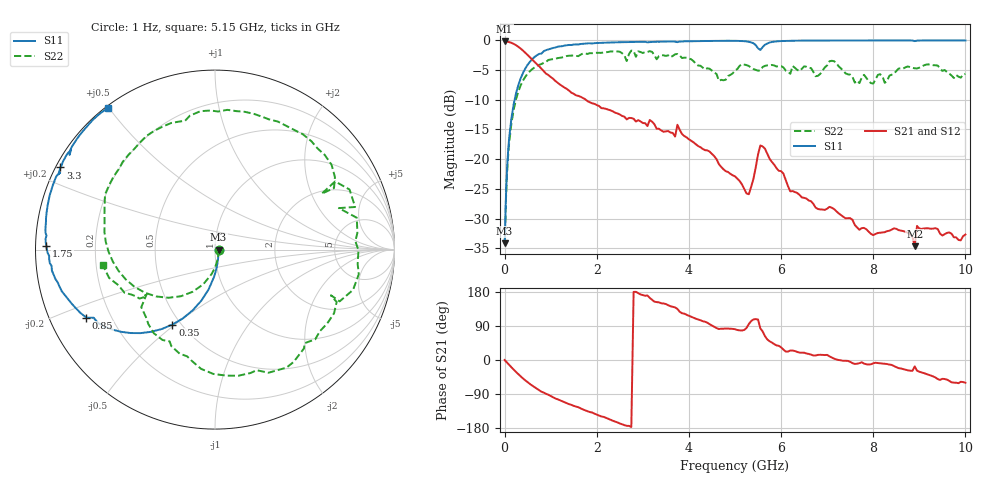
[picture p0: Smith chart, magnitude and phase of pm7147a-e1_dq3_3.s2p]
# GHz S DB R 50
! S-Parameters data
! Freq  dbS11  angS11  dbS21  angS21  dbS12  angS12  dbS22  angS22
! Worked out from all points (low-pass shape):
!   279 points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, 1 Hz to 10 GHz, reference 50 ohm
!   highest |S21| = -0.17 dB at 19.95 kHz (marker M1); lowest = -34.7 dB at 8.9 GHz (marker M2)
!   |S21| within 3 dB of the highest: start of sweep to 592.2 MHz
!   lowest |S11| = -34.2 dB at 19.95 kHz (marker M3), VSWR 1.04, Z = 52 - j0.00267 ohm
!   |S11| at or under -10 dB: start of sweep to 217.4 MHz
!   |S22| runs from -34.2 to -1.7 dB; largest |S21 - S12| = 0
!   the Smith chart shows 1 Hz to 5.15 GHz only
!   S11 on the Smith chart (normalised r, x): 1 Hz: 1.04, -0.00; 350 MHz: 0.45, -0.49; 850 MHz: 0.11, -0.24; 1.75 GHz: 0.03, +0.01; 3.3 GHz: 0.01, +0.25; 5.15 GHz: 0.01, +0.50
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1e-09  -34.18 -0.0  -0.17 -0.0  -0.17 -0.0  -34.18 -0.0
1.99526e-05  -34.18 -0.1  -0.17 -0.0  -0.17 -0.0  -34.18 -0.1
0.1  -16.36 -92.0  -0.28 -13.0  -0.28 -13.0  -17.19 -98.0
0.35  -6.37 -119.6  -1.39 -43.3  -1.39 -43.3  -7.55 -141.5
0.85  -1.82 -152.2  -5.20 -86.1  -5.20 -86.1  -3.78 162.1
1.7  -0.57 179.9  -9.71 -130.5  -9.71 -130.5  -2.21 96.1
1.75  -0.54 178.8  -9.92 -133.0  -9.92 -133.0  -2.21 91.8
2.8  -0.26 159.2  -13.19 179.8  -13.19 179.8  -1.77 16.9
3.3  -0.22 152.0  -14.87 152.8  -14.87 152.8  -3.17 -21.5
3.35  -0.22 151.2  -14.88 152.1  -14.88 152.1  -2.64 -23.3
4  -0.14 142.8  -16.64 116.8  -16.64 116.8  -3.04 -85.0
5.05  -0.08 128.8  -23.27 79.2  -23.27 79.2  -4.83 -159.8
5.15  -0.10 127.2  -24.24 77.8  -24.24 77.8  -3.98 -172.4
5.3  -0.23 124.3  -25.90 94.9  -25.90 94.9  -4.31 170.1
5.55  -1.62 125.3  -17.70 83.5  -17.70 83.5  -5.05 156.7
6  -0.11 122.9  -22.02 33.5  -22.02 33.5  -4.33 119.8
6.7  -0.02 115.1  -27.54 11.9  -27.54 11.9  -5.29 78.8
7.05  -0.01 111.8  -28.03 9.6  -28.03 9.6  -3.51 72.3
8.35  -0.01 101.0  -32.04 -12.1  -32.04 -12.1  -5.95 28.8
8.9  -0.11 96.1  -34.65 -16.9  -34.65 -16.9  -4.69 -3.6
8.95  -0.03 97.2  -31.24 -28.0  -31.24 -28.0  -4.72 -5.0
10  -0.01 89.9  -32.69 -59.9  -32.69 -59.9  -5.65 -59.7
